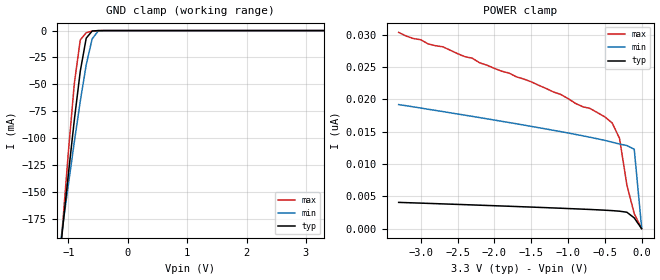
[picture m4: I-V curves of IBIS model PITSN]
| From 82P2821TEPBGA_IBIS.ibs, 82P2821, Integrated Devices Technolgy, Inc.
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|   Model PITSN
[Model]		PITSN
Model_type	Input
Polarity   Non-Inverting
Vinl = 		0.8000V
Vinh = 		2.0000V
C_comp   4.8700pF   4.2900pF   5.3700pF
[Temperature Range]	  25.0000   90.0000   -40.0000
[Voltage Range]   3.3000V   3.0000V   3.6000V
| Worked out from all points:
|   GND clamp passes 1 mA (typ) near -0.61 V on its own axis
[GND_clamp]
|Voltage	  I(typ)   I(min)   I(max)
-3.3V     -1.417A    -1.129A    -1.858A
-1.2V     -239.2mA   -225mA     -255.1mA
-1.1V     -185.7mA   -183.7mA   -182.6mA
-1V       -133.3mA   -143.1mA   -112.7mA
-900mV    -83.06mA   -103.5mA   -49.1mA
-800mV    -37.76mA   -65.72mA   -8.671mA
-700mV    -7.074mA   -31.79mA   -2.029mA
-600mV    -432.4uA   -7.705mA   -441uA
-500mV    -28.08uA   -555.9uA   -48.67uA
3.3V      871.2fA    13.1nA     -671.3pA
[POWER_clamp]
|Voltage	  I(typ)   I(min)   I(max)
-3.3V     4.069nA    19.21nA    30.39nA
-2.9V     3.915nA    18.49nA    28.61nA
-2.7V     3.835nA    18.13nA    28.16nA
-2.2V     3.635nA    17.2nA     25.68nA
-1.5V     3.343nA    15.84nA    22.74nA
-1.1V     3.165nA    15.03nA    20.79nA
-500mV    2.86nA     13.67nA    17.31nA
-400mV    2.794nA    13.39nA    16.37nA
-300mV    2.707nA    13.1nA     13.99nA
-200mV    2.543nA    12.87nA    6.768nA
-100mV    1.667nA    12.3nA     2.315nA
0V        871.7fA    200.7pA    631.4fA
